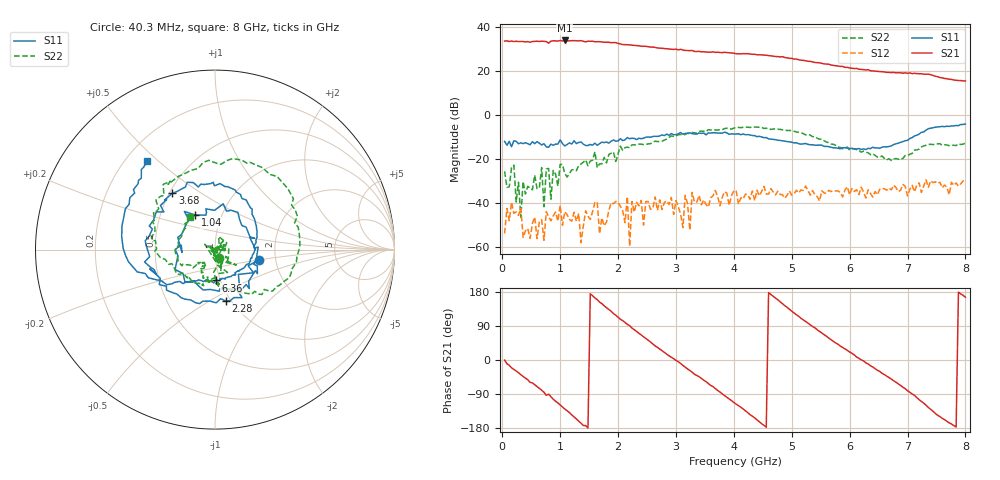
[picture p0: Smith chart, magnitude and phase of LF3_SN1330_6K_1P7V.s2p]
! VC=1.7V I=9.98mA
# HZ S DB R 50.00
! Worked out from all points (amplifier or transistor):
!   200 points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, 40.3 MHz to 8 GHz, reference 50 ohm
!   highest |S21| = 33.8 dB at 1.08 GHz (marker M1)
!   |S21| within 3 dB of that: start of sweep to 2.552 GHz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
!   unconditionally stable (mu >= 1): start of sweep to 3.679 GHz; 4.048 GHz to 4.317 GHz; 4.527 GHz to end of sweep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
!   at 1.36 GHz: K = 7.62, MAG = 34.0 dB, |S12| = -57.9 dB
!   at 4.04 GHz: K = 0.94, MSG = 31.0 dB, |S12| = -34.3 dB
!   at 8 GHz: K = 1.67, MAG = 17.6 dB, |S12| = -29.5 dB
!   S11 on the Smith chart (normalised r, x): 40.3 MHz: 1.63, -0.20; 1.04 GHz: 0.75, +0.30; 2.28 GHz: 0.95, -0.59; 3.68 GHz: 0.52, +0.38; 6.36 GHz: 0.95, -0.34; 8 GHz: 0.29, +0.46
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4.02985e7  -12.00 -13.5  33.52 -0.3  -53.77 83.3  -25.61 -67.7
1.60294e8  -14.44 -46.7  33.50 -20.7  -39.65 54.1  -23.89 152.4
6.002775e8  -12.10 -153.5  33.44 -70.1  -56.12 -34.9  -33.45 43.0
8.80267e8  -13.78 155.4  33.63 -103.5  -45.81 75.6  -25.15 -5.7
1.040261e9  -13.03 120.0  33.53 -124.0  -50.06 92.4  -22.50 29.1
1.08026e9  -14.05 104.9  33.78 -129.3  -43.86 149.4  -26.57 -5.6
1.400248e9  -13.26 51.0  33.43 -173.0  -50.33 112.0  -21.41 -28.7
1.640238e9  -13.77 19.4  33.22 159.4  -39.48 -16.9  -23.96 -72.9
1.920228e9  -11.31 -29.6  32.79 122.4  -40.30 -76.8  -16.77 -61.2
2.280214e9  -10.67 -77.9  31.51 80.0  -44.08 8.9  -13.56 -107.3
2.720198e9  -9.56 -133.2  30.30 28.9  -38.55 -71.2  -12.10 -157.7
3.080184e9  -7.99 -170.0  29.79 -9.1  -44.97 -139.9  -8.87 169.4
3.680162e9  -8.09 127.2  28.36 -75.5  -34.28 -157.7  -6.81 116.4
4.040148e9  -8.67 93.6  27.75 -116.3  -34.33 -170.4  -5.75 79.1
4.560129e9  -10.26 47.6  27.10 -177.3  -35.88 126.7  -6.05 26.3
5.000112e9  -12.40 15.0  25.63 129.0  -36.42 94.7  -7.07 -20.6
5.360099e9  -13.54 -13.0  24.07 88.5  -34.31 65.0  -9.86 -46.4
5.88008e9  -14.91 -49.9  21.99 33.1  -37.23 31.7  -15.34 -96.7
6.360062e9  -15.28 -88.9  20.06 -15.4  -35.55 -1.3  -18.04 -125.1
6.68005e9  -14.33 -118.6  19.29 -46.7  -33.17 -36.0  -19.86 -125.8
7.400022e9  -6.04 -176.0  18.26 -130.4  -29.87 -94.8  -13.31 -161.9
8e9  -4.15 127.5  15.39 165.7  -29.46 -138.4  -12.83 127.6
